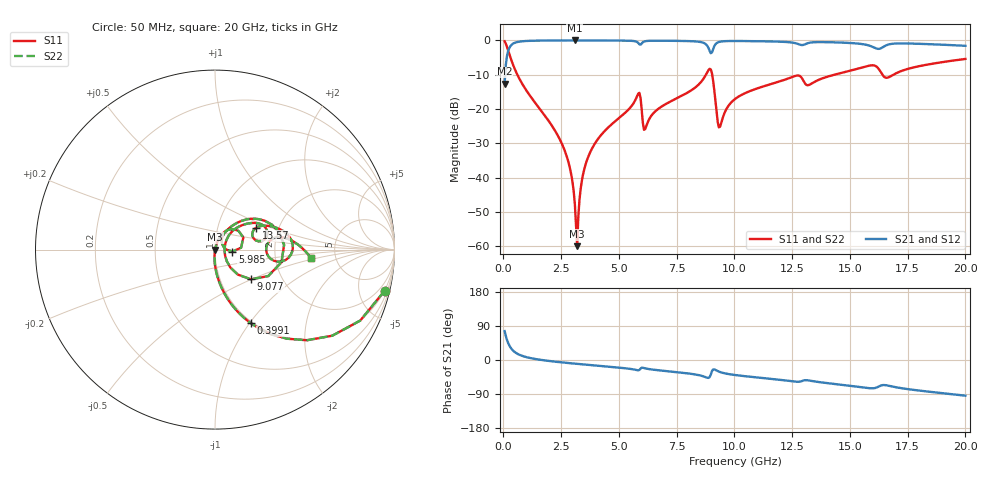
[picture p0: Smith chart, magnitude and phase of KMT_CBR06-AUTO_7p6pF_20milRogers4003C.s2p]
! Data measured by Modelithics Inc. support@modelithics.com 813-866-6335
! KEMET CBR06-AUTO 7.6pF, Pad Width= 0.851mm, Pad Length= 0.64mm, Pad Gap= 0.62mm, 20mil Rogers 4003C substrate Data, January 2022
# hz S ma R 50
! 2 Port Network Data from SP1.SP block
! freq  magS11  angS11  magS21  angS21  magS12  angS12  magS22  angS22
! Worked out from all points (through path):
!   401 points, 50 MHz to 20 GHz, reference 50 ohm
!   highest |S21| = -0.01 dB at 3.092 GHz (marker M1); lowest = -12.6 dB at 50 MHz (marker M2)
!   group delay of S21, straight-line fit = 14.3 ps
!   lowest |S11| = -60.0 dB at 3.192 GHz (marker M3), VSWR 1.00, Z = 50.1 + j0.0234 ohm
!   |S11| at or under -10 dB: 601.7 MHz to 8.767 GHz (8.165 GHz wide, 174 % of centre); 9.037 GHz to 14.33 GHz (5.292 GHz wide, 45.3 % of centre); 16.41 GHz to 16.88 GHz (477.8 MHz wide, 2.87 % of centre)
!   |S22| runs from -60.0 to -0.2 dB; largest |S21 - S12| = 0
!   S11 on the Smith chart (normalised r, x): 50 MHz: 0.98, -8.21; 399.1 MHz: 0.98, -1.01; 5.985 GHz: 1.22, -0.03; 9.077 GHz: 1.40, -0.50; 13.57 GHz: 1.53, +0.40; 20 GHz: 3.26, -0.43
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5e7  0.9722 -13.7  0.234 76.3  0.234 76.3  0.9722 -13.7
3.99125e8  0.456 -64.1  0.8894 25.9  0.8894 25.9  0.456 -64.1
2.54375e9  0.03042 -94.8  0.9986 -6.4  0.9986 -6.4  0.03042 -94.8
2.892875e9  0.01304 -94.7  0.9989 -8.5  0.9989 -8.5  0.01304 -94.7
3.092375e9  0.004047 -86.8  0.999 -9.6  0.999 -9.6  0.004047 -86.8
3.192125e9  0.0009986 13.5  0.999 -10.2  0.999 -10.2  0.0009986 13.5
3.391625e9  0.008858 72.5  0.9989 -11.3  0.9989 -11.3  0.008858 72.5
4.2395e9  0.04218 72.5  0.9978 -15.9  0.9978 -15.9  0.04218 72.5
5.785625e9  0.1538 47.7  0.948 -26.9  0.948 -26.9  0.1538 47.7
5.985125e9  0.09784 -6.5  0.9045 -20.4  0.9045 -20.4  0.09784 -6.5
6.13475e9  0.05074 37.6  0.9731 -22.0  0.9731 -22.0  0.05074 37.6
6.73325e9  0.1023 60.3  0.9902 -27.2  0.9902 -27.2  0.1023 60.3
8.678375e9  0.2818 37.6  0.9172 -43.6  0.9172 -43.6  0.2818 37.6
9.077375e9  0.2598 -39.6  0.7462 -24.9  0.7462 -24.9  0.2598 -39.6
9.376625e9  0.05506 11.5  0.9589 -31.8  0.9589 -31.8  0.05506 11.5
1.0025e10  0.1397 46.7  0.9809 -39.6  0.9809 -39.6  0.1397 46.7
1.266838e10  0.3058 24.1  0.9071 -57.3  0.9071 -57.3  0.3058 24.1
1.336662e10  0.2377 26.3  0.9374 -55.5  0.9374 -55.5  0.2377 26.3
1.356612e10  0.2586 28.0  0.9448 -57.4  0.9448 -57.4  0.2586 28.0
1.591025e10  0.4327 4.7  0.8247 -74.7  0.8247 -74.7  0.4327 4.7
1.670825e10  0.2933 5.9  0.8788 -68.3  0.8788 -68.3  0.2933 5.9
2e10  0.5373 -5.0  0.8346 -94.2  0.8346 -94.2  0.5373 -5.0
